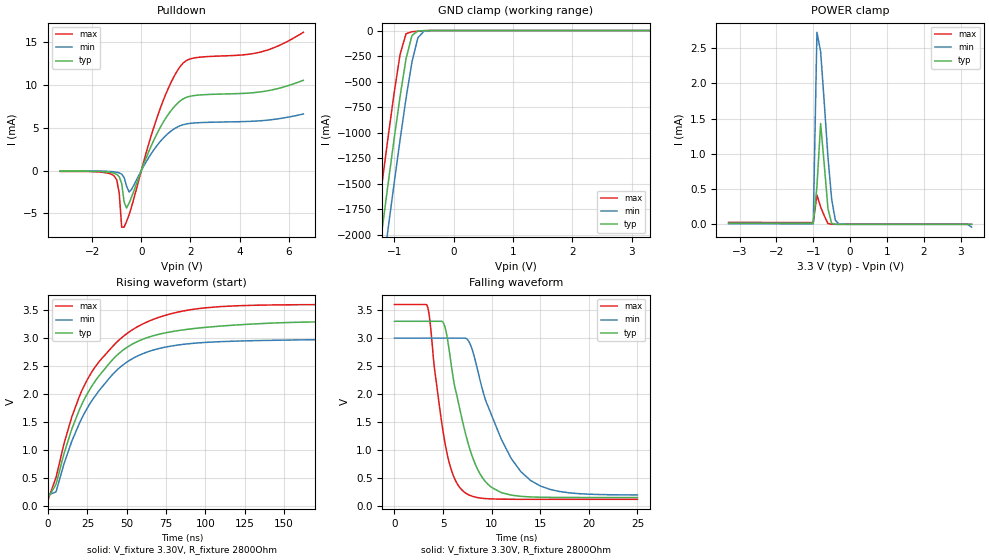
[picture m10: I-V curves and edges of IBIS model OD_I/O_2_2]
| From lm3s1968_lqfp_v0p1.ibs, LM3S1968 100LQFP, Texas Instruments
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[Model]   OD_I/O_2_2
Model_type   I/O_open_drain
Polarity   Inverting
Vinl = 1.26
Vinh = 2.04
Vmeas = 1.65
Rref = 2800
Vref = 3.3
| variable   typ   min   max
C_comp   9.739pF   9.739pF   9.739pF
[Model Spec]
Vinh+   1.91   1.78   2.04
Vinh-   1.90   1.76   2.03
Vinl+   1.40   1.27   1.54
Vinl-   1.39   1.26   1.53
| variable   typ   min   max
[Temperature Range]  25   85   -40
[Voltage Range]   3.3V   3.0V   3.6V
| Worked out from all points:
|   slope of the pulldown table from 0 to 0.495 V, typ, clamps not added: 143 ohm
|   GND clamp passes 1 mA (typ) near -0.48 V on its own axis
|   POWER clamp passes 1 mA (typ) near -0.73 V on its own axis
|   falling waveform, V_fixture 3.30V, R_fixture 2800Ohm: 20-80 % time 2.51ns typ, 3.85ns min, 1.7ns max; typ from 3.3 V to 0.149 V
|   rising waveform, V_fixture 3.30V, R_fixture 2800Ohm: 20-80 % time 34.2ns typ, 33.9ns min, 35.2ns max; typ from 0.149 V to 3.3 V
[Pulldown]
|  Voltage   I(typ)   I(min)   I(max)
-3.3V     -64.15uA   -36.41uA   -91.13uA
-1.1V     -318.3uA   -146.9uA   -641.8uA
-900mV    -721.3uA   -265.2uA   -2.635mA
-800mV    -1.498mA   -417.6uA   -6.598mA
-700mV    -3.678mA   -803.7uA   -6.582mA
-600mV    -4.358mA   -1.83mA    -5.933mA
-500mV    -3.814mA   -2.5mA     -5.165mA
700mV     4.654mA    3.152mA    6.687mA
1.2V      6.961mA    4.59mA     10.23mA
1.7V      8.361mA    5.354mA    12.53mA
4.9V      9.201mA    5.826mA    13.87mA
6.6V      10.54mA    6.604mA    16.13mA
[GND Clamp]
|  Voltage   I(typ)   I(min)   I(max)
-3.3V     -11.72A    -12.12A    -11.3A
-1.4V     -2.845A    -3.285A    -2.387A
-1.3V     -2.39A     -2.831A    -1.93A
-1.2V     -1.938A    -2.38A     -1.478A
-1.1V     -1.494A    -1.934A    -1.036A
-1V       -1.059A    -1.496A    -610.6mA
-900mV    -645mA     -1.069A    -232.9mA
-800mV    -277.1mA   -664.4mA   -31.59mA
-700mV    -48.56mA   -306.6mA   -12.09mA
-600mV    -5.558mA   -70.2mA    -6.272mA
-500mV    -1.167mA   -7.88mA    -2.167mA
3.3V      2.282nA    3.101uA    451.3pA
[POWER Clamp]
|  Voltage   I(typ)   I(min)   I(max)
-3.3V     15.18uA    8.315uA    27.48uA
-1V       14.14uA    7.74uA     25.63uA
-900mV    536uA      2.726mA    416.7uA
-800mV    1.43mA     2.454mA    247.6uA
-700mV    840.7uA    1.719mA    119.9uA
-600mV    221.2uA    951.5uA    11.58uA
-500mV    12.35uA    355.6uA    955.3nA
-400mV    305.2nA    58.59uA    44.3nA
-300mV    9.515nA    3.101uA    1.472nA
3.1V      1.302nA    -112.7nA   143.5pA
3.2V      1.207nA    -2.287uA   131.7pA
3.3V      -104.8pA   -40.34uA   119.2pA
[Ramp]
| variable   typ   min   max
dV/dt_f   1.89/2.51n   1.68/3.85n   2.09/1.70n
dV/dt_r   1.89/34.25n   1.68/33.89n   2.09/35.24n
R_load = 2800Ohm
[Falling Waveform]
V_fixture = 3.30V
V_fixture_min = 3.00V
V_fixture_max = 3.60V
R_fixture = 2800Ohm
|   Time   V(typ)   V(min)   V(max)
0s        3.3V       2.999V     3.6V
3.4ns     3.3V       2.999V     3.567V
5.3ns     3.125V     2.999V     1.033V
6.1ns     2.23V      2.999V     523.5mV
7.2ns     1.369V     2.999V     244.6mV
7.9ns     937mV      2.845V     178mV
9.3ns     446.7mV    1.93V      131.1mV
13ns      169.9mV    611.5mV    117mV
17ns      150.3mV    255.8mV    116.6mV
25ns      149mV      194.8mV    116.5mV
[Rising Waveform]
V_fixture = 3.30V
V_fixture_min = 3.00V
V_fixture_max = 3.60V
R_fixture = 2800Ohm
|   Time   V(typ)   V(min)   V(max)
0s        148.8mV    194.4mV    116.4mV
5ns       383mV      248.9mV    506.6mV
10ns      925.9mV    744.5mV    1.104V
15ns      1.371V     1.153V     1.587V
25ns      2.01V      1.753V     2.26V
43ns      2.672V     2.407V     2.908V
60ns      2.976V     2.718V     3.249V
82ns      3.13V      2.873V     3.46V
110ns     3.214V     2.936V     3.562V
250ns     3.298V     2.994V     3.599V
